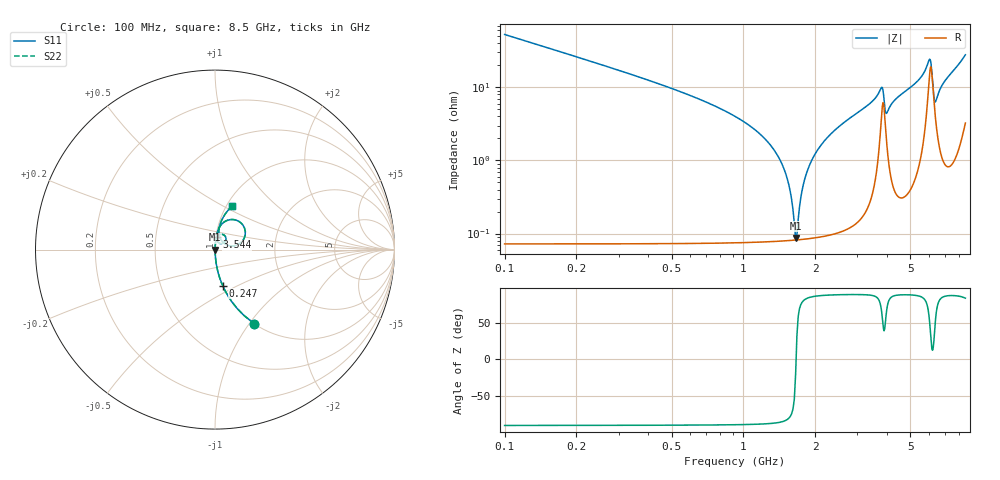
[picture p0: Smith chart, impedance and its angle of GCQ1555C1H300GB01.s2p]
!Murata Part Number: GCQ1555C1H300GB01
!These Parameters are Measured in Series Mode Connection
!Data Generated on Mar 13, 2026
!  o--ll--o
!Port1  Port2
!  o------o
!Operation Temp=25[degC], DC Bias Voltage=0[V]
!Freq. Start=100[MHz] Stop=9[GHz] 401[Steps]
# Hz S RI R 50
!Freq.(Hz) S11(Real) S11(Imag) S21(Real) S21(Imag) S12(Real) S12(Imag) S22(Real) S22(Imag)
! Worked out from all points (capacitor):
!   401 points, 100 MHz to 8.5 GHz, reference 50 ohm
!   read as one part in series: C = 30 pF near 142 MHz
!   lowest |Z| = 86.8 mohm at 1.654 GHz (marker M1)
!   series resonance near 1.662 GHz, so ESL is about 310 pH
!   S11 on the Smith chart (normalised r, x): 100 MHz: 1.00, -1.06; 247 MHz: 1.00, -0.42; 3.544 GHz: 1.01, +0.14; 8.5 GHz: 1.06, +0.55
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1e8  0.2187 -0.4127  0.7813 0.4127  0.7813 0.4127  0.2187 -0.4127
2.47e8  0.0429 -0.201  0.9571 0.201  0.9571 0.201  0.0429 -0.201
4.99e8  0.01 -0.0959  0.99 0.0959  0.99 0.0959  0.01 -0.0959
1.234e9  0.00115 -0.0195  0.9989 0.0195  0.9989 0.0195  0.00115 -0.0195
1.507e9  0.000835 -0.00636  0.9992 0.00636  0.9992 0.00636  0.000835 -0.00636
1.654e9  0.000814 -0.000299  0.9992 0.000299  0.9992 0.000299  0.000814 -0.000299
1.696e9  0.000821 0.00134  0.9992 -0.00134  0.9992 -0.00134  0.000821 0.00134
1.759e9  0.000843 0.00374  0.9992 -0.00374  0.9992 -0.00374  0.000843 0.00374
1.822e9  0.000876 0.00607  0.9991 -0.00607  0.9991 -0.00607  0.000876 0.00607
2.011e9  0.00104 0.0127  0.999 -0.0127  0.999 -0.0127  0.00104 0.0127
2.368e9  0.00157 0.0244  0.9984 -0.0244  0.9984 -0.0244  0.00157 0.0244
2.914e9  0.00305 0.0417  0.9969 -0.0417  0.9969 -0.0417  0.00305 0.0417
3.544e9  0.00954 0.0684  0.9905 -0.0684  0.9905 -0.0684  0.00954 0.0684
3.796e9  0.0501 0.0812  0.9499 -0.0812  0.9499 -0.0812  0.0501 0.0812
3.964e9  0.0215 0.0373  0.9785 -0.0373  0.9785 -0.0373  0.0215 0.0373
4.3e9  0.00815 0.0659  0.9918 -0.0659  0.9918 -0.0659  0.00815 0.0659
5.707e9  0.0439 0.1483  0.9561 -0.1483  0.9561 -0.1483  0.0439 0.1483
6.043e9  0.1645 0.1198  0.8355 -0.1198  0.8355 -0.1198  0.1645 0.1198
6.274e9  0.0632 0.0277  0.9368 -0.0277  0.9368 -0.0277  0.0632 0.0277
6.358e9  0.0408 0.045  0.9592 -0.045  0.9592 -0.045  0.0408 0.045
7.114e9  0.0251 0.1285  0.9749 -0.1285  0.9749 -0.1285  0.0251 0.1285
8.5e9  0.0964 0.2423  0.9036 -0.2423  0.9036 -0.2423  0.0964 0.2423
